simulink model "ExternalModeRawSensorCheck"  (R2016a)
settings: Solver=FixedStepAuto  StartTime=0.0  StopTime=inf  RelTol=1e-3
libraries: miniQ x1

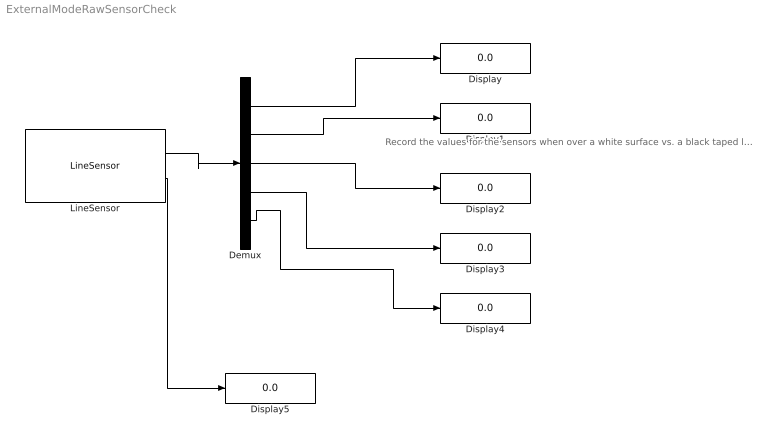
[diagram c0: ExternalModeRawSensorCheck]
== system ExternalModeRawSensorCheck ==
  note: Record the values for the sensors when over a white surface vs. a black taped line. Identify a large "threshold" drop in the values when moving from one color to another.
  Demux : Demux  Outputs=5
  Display{,1..5} (6 alike) : Display
  LineSensor : miniQ/LineSensor  sampleTime_dd=0.01  maxRawSensors=[800,900,900,900,800]  minRawSensors=[200,280,300,300,220]  debug_dd=off
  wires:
  LineSensor/2 -> Display5/1
  Demux/1 -> Display/1
  LineSensor/1 -> Demux/1
  Demux/4 -> Display3/1
  Demux/2 -> Display1/1
  Demux/5 -> Display4/1
  Demux/3 -> Display2/1
